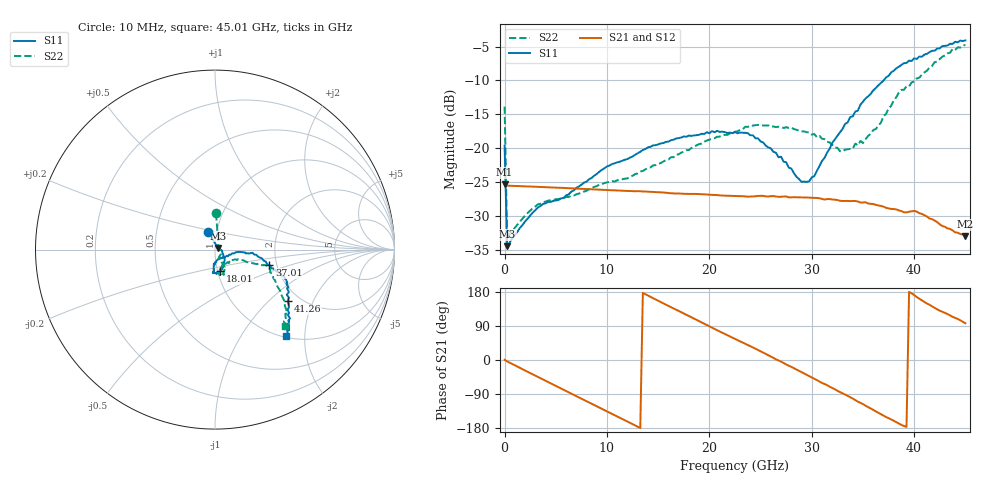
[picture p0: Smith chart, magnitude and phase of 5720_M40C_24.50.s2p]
! Device:  ADRF5720
! Description: 0.5dB LSB GaAs MMIC 6-bit Digital Attenuator
! Frequency:  0.000009 -  40 GHz
! Ports:
!	RF1	= Port 1
!	RF2	= Port 2
! Vdd:  3.3 Volt
! Vss:  -3.3 Volt
! Control:  0/3.3 Volt
! State:  24.50 dB attenuation
! Data:  The device was measured using G-S-G Probes on a matrix board.
!  Data was collected using an calibrated 4 port network analyzer.
!  The reference plane for this measurement is at the launchers.
! Note:  Analog Devices supplies this data as a sample of measured data
!  for this product.  Your particular data for this product may vary.
!  Data was taken at -40 degrees C.
!  Analog Devices reserves the right to change this data at anytime.
# GHZ S DB R 45.0
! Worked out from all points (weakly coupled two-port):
!   181 points, 10 MHz to 45.01 GHz, reference 45 ohm
!   highest |S21| = -25.36 dB at 10 MHz (marker M1); lowest = -33.0 dB at 45.01 GHz (marker M2)
!   lowest |S11| = -34.5 dB at 260 MHz (marker M3), VSWR 1.04, Z = 46.5 + j0.896 ohm
!   |S11| at or under -10 dB: start of sweep to 37.03 GHz
!   |S22| runs from -33.4 to -4.8 dB; largest |S21 - S12| = 0.00023
!   S11 on the Smith chart (normalised r, x): 10 MHz: 0.91, +0.18; 18.01 GHz: 1.03, -0.25; 37.01 GHz: 1.83, -0.35; 41.26 GHz: 1.72, -1.32; 45.01 GHz: 1.02, -1.61
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0.01  -19.64 111.1  -25.36 0.4  -25.38 0.4  -13.87 88.3
0.26  -34.47 30.6  -25.54 -3.7  -25.56 -3.8  -33.42 22.5
3.26  -28.76 -5.7  -25.72 -44.7  -25.74 -44.7  -28.31 -29.3
5.76  -27.36 -19.7  -25.87 -78.4  -25.90 -78.4  -27.40 -48.6
7.76  -25.09 -33.4  -26.02 -105.3  -26.03 -105.3  -26.41 -61.9
10.01  -22.69 -43.3  -26.18 -135.6  -26.20 -135.7  -25.06 -65.8
15.26  -19.30 -65.4  -26.52 152.9  -26.54 152.8  -22.19 -62.0
18.01  -18.13 -76.5  -26.76 116.1  -26.78 116.0  -20.27 -60.7
22.76  -17.80 -94.4  -27.08 52.4  -27.10 52.3  -17.51 -69.1
24.76  -18.55 -93.1  -27.05 26.3  -27.07 26.2  -16.57 -71.3
27.01  -21.26 -91.7  -27.17 -4.4  -27.19 -4.5  -16.89 -78.2
29.01  -24.96 -73.3  -27.27 -32.0  -27.30 -32.1  -17.52 -81.4
30.26  -24.12 -41.0  -27.34 -49.4  -27.36 -49.6  -17.92 -79.9
33.01  -17.19 -5.3  -27.80 -87.5  -27.82 -87.7  -20.50 -59.4
35.01  -13.14 -7.2  -28.03 -116.5  -28.05 -116.6  -19.24 -32.9
37.01  -10.04 -15.8  -28.63 -146.9  -28.66 -147.0  -15.27 -20.6
37.76  -8.82 -19.5  -28.97 -156.8  -28.99 -156.9  -13.75 -20.5
38.76  -7.72 -21.2  -29.29 -171.2  -29.30 -171.5  -11.40 -18.8
39.76  -7.13 -25.4  -29.33 175.9  -29.34 175.7  -10.29 -17.0
41.26  -6.07 -35.4  -30.10 148.9  -30.12 149.0  -8.56 -26.9
43.76  -4.60 -45.7  -32.14 113.9  -32.17 113.6  -5.36 -41.5
45.01  -4.10 -50.6  -32.99 97.1  -33.03 96.9  -4.78 -47.5
